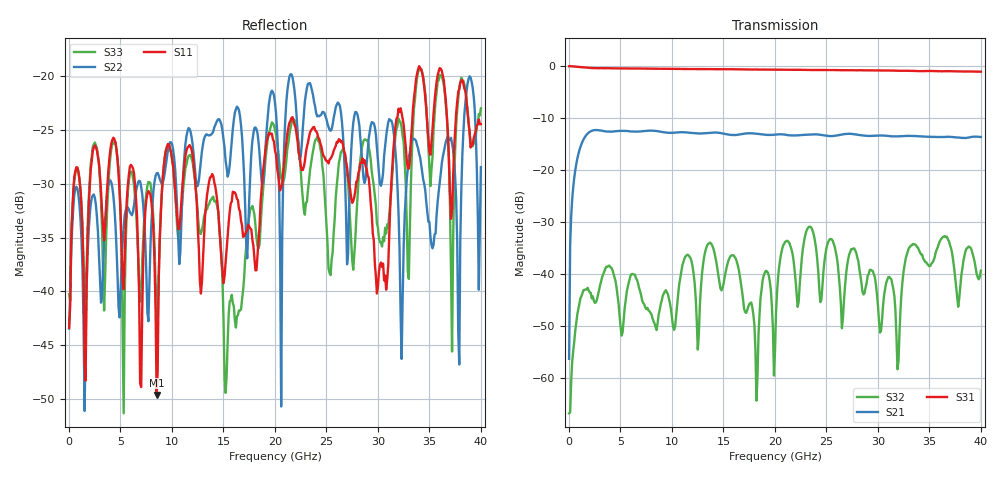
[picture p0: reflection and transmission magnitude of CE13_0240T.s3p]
!Keysight Technologies,N5245A,MY52451697,A.10.60.06
!Date: Thursday, December 02, 2021 17:48:07
!Correction: S11(Full 4 Port(1,2,3,4))
!S13(Full 4 Port(1,2,3,4))
!S14(Full 4 Port(1,2,3,4))
!S31(Full 4 Port(1,2,3,4))
!S33(Full 4 Port(1,2,3,4))
!S34(Full 4 Port(1,2,3,4))
!S41(Full 4 Port(1,2,3,4))
!S43(Full 4 Port(1,2,3,4))
!S44(Full 4 Port(1,2,3,4))
!S3P File: Measurements: <S11,S13,S14>,
!<S31,S33,S34>,
!<S41,S43,S44>:
# Hz S  dB  R 50
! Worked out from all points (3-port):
!   401 points, 10 MHz to 40 GHz, reference 50 ohm
!   strongest paths, dB at 10 MHz, 10.01 GHz, 20 GHz, 30 GHz, 40 GHz:
!     S31: 0.0, -0.5, -0.7, -0.8, -1.1
!     S21: -56.4, -12.9, -13.2, -13.4, -13.7
!     S32: -66.9, -48.6, -54.8, -46.1, -39.4
!   lowest |S11| = -49.6 dB at 8.508 GHz (marker M1), VSWR 1.01, Z = 49.9 - j0.301 ohm
!   |S11| at or under -10 dB: start of sweep to end of sweep
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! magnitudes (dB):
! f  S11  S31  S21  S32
! 10 MHz  -43.4  0.0  -56.4  -66.9
! 1.41 GHz  -38.3  -0.3  -14.1  -43.1
! 8.508 GHz  -49.6  -0.5  -12.5  -50.8
! 13.71 GHz  -29.4  -0.6  -12.9  -34.0
! 15.31 GHz  -36.2  -0.6  -13.1  -38.8
! 20 GHz  -26.9  -0.7  -13.2  -54.8
! 23.3 GHz  -25.7  -0.8  -13.2  -30.9
! 31.9 GHz  -23.8  -0.9  -13.5  -58.4
! 33.2 GHz  -26.0  -0.9  -13.5  -34.6
! 40 GHz  -24.5  -1.1  -13.7  -39.4
